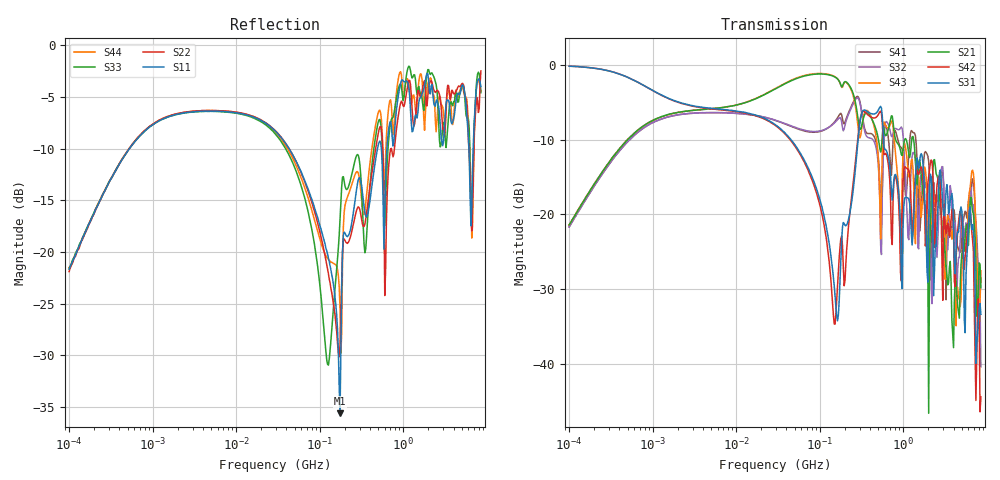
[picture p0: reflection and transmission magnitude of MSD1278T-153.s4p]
# MHz S MA R 50
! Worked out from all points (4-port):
!   498 points, 100 kHz to 8.5 GHz, reference 50 ohm
!   strongest paths, dB at 100 kHz, 1.698 MHz, 29.49 MHz, 500.7 MHz, 8.5 GHz:
!     S31: -0.2, -4.6, -8.0, -6.1, -33.4
!     S42: -0.2, -4.7, -8.1, -6.7, -44.4
!     S21: -21.4, -6.5, -3.2, -9.8, -29.8
!     S43: -21.4, -6.5, -3.1, -12.3, -27.5
!     S32: -21.7, -6.8, -7.4, -13.2, -40.4
!     S41: -21.6, -6.8, -7.4, -12.1, -29.1
!   lowest |S11| = -35.6 dB at 175.1 MHz (marker M1), VSWR 1.03, Z = 51.7 + j0.226 ohm
!   |S11| at or under -10 dB: 42.95 MHz to 492.1 MHz (449.2 MHz wide, 168 % of centre); 546.4 MHz to 637.4 MHz (91.03 MHz wide, 15.4 % of centre); 6.109 GHz to 6.879 GHz (770.2 MHz wide, 11.9 % of centre)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
0.1  0.08266 77.6  0.08513 78.6  0.9811 -4.9  0.08272 -101.9
     0.08513 78.6  0.08033 78.8  0.08242 -101.9  0.9817 -4.9
     0.9811 -4.9  0.08242 -101.9  0.08271 78.7  0.08502 78.4
     0.08272 -101.9  0.9817 -4.9  0.08502 78.4  0.08409 79.4
14.8634  0.4546 -18.5  0.5758 12.8  0.4725 -26.0  0.4644 155.2
         0.5758 12.8  0.4577 -20.1  0.4654 153.6  0.4677 -26.2
         0.4725 -26.0  0.4654 153.6  0.4505 -20.3  0.5774 12.7
         0.4644 155.2  0.4677 -26.2  0.5774 12.7  0.4559 -18.4
175.1055  0.01657 7.6  0.7586 -47.3  0.03636 -76.5  0.4717 34.0
          0.7586 -47.3  0.03527 -177.6  0.4446 25.8  0.06098 38.7
          0.03636 -76.5  0.4446 25.8  0.1427 58.5  0.7574 -53.0
          0.4717 34.0  0.06098 38.7  0.7574 -53.0  0.05294 -24.7
524.0594  0.3439 8.8  0.2767 -89.2  0.5222 -72.7  0.164 -95.0
          0.2767 -89.2  0.4026 -0.2  0.1264 -103.2  0.4865 -76.6
          0.5222 -72.7  0.1264 -103.2  0.4379 -9.9  0.1213 -128.8
          0.164 -95.0  0.4865 -76.6  0.1213 -128.8  0.4857 -6.2
1113.489  0.6692 -117.9  0.3005 -152.3  0.1294 -148.8  0.1615 6.6
          0.3005 -152.3  0.6181 -94.4  0.09834 115.1  0.2023 -139.9
          0.1294 -148.8  0.09834 115.1  0.7496 -107.6  0.2292 -164.0
          0.1615 6.6  0.2023 -139.9  0.2292 -164.0  0.69 -114.4
2159.325  0.6366 -179.3  0.1105 170.6  0.1783 111.1  0.0366 -3.1
          0.1105 170.6  0.6742 -175.4  0.03345 60.5  0.2316 111.7
          0.1783 111.1  0.03345 60.5  0.7343 140.2  0.08616 142.1
          0.0366 -3.1  0.2316 111.7  0.08616 142.1  0.6891 171.3
8500  0.631 -57.9  0.03235 -108.4  0.02149 -112.5  0.03528 176.0
      0.03235 -108.4  0.7511 -39.0  0.009571 147.2  0.006022 178.9
      0.02149 -112.5  0.009571 147.2  0.5895 -54.0  0.04202 -61.2
      0.03528 176.0  0.006022 178.9  0.04202 -61.2  0.6007 -60.1
